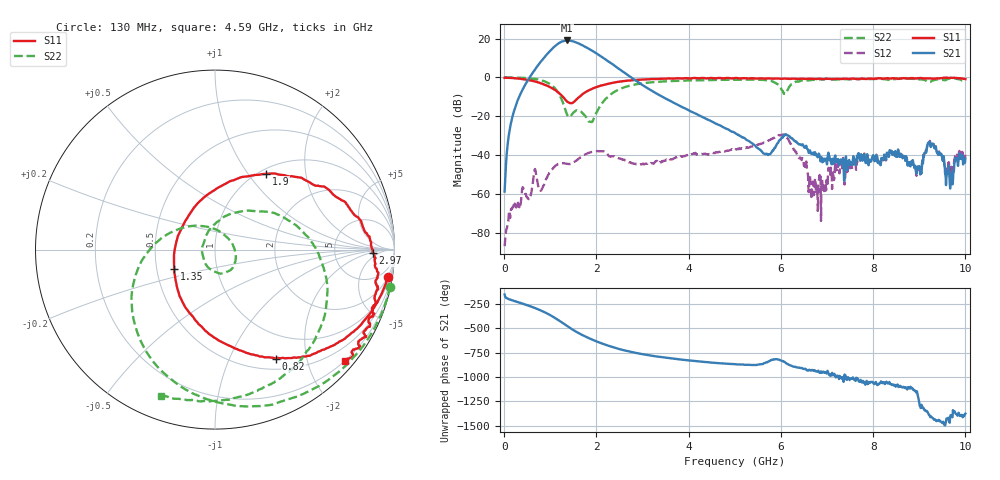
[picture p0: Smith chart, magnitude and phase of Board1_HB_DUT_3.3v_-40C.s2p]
! Created Tue May 27 11:37:13 2025
# hz S ma R 50
! 2 Port Network Data from SP1.SP block
! freq  magS11  angS11  magS21  angS21  magS12  angS12  magS22  angS22
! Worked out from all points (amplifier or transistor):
!   1000 points, 10 MHz to 10 GHz, reference 50 ohm
!   highest |S21| = 19.0 dB at 1.36 GHz (marker M1)
!   |S21| within 3 dB of that: 1.097 GHz to 1.738 GHz (640.7 MHz wide, 45.2 % of centre)
!   unconditionally stable (mu >= 1): 19.38 MHz to 24.58 MHz; 87.49 MHz to 108.8 MHz; 111.2 MHz to end of sweep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
!   at 1.67 GHz: K = 6.85, MAG = 17.5 dB, |S12| = -40.8 dB
!   at 5.01 GHz: K = 11.66, MAG = -9.4 dB, |S12| = -37.1 dB
!   at 10 GHz: K = 402.10, MAG = -30.0 dB, |S12| = -39.7 dB
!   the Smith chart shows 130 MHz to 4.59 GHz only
!   S11 on the Smith chart (normalised r, x): 130 MHz: 2, -12; 820 MHz: 0.64, -1.51; 1.35 GHz: 0.62, -0.14; 1.9 GHz: 1.08, +1.23; 2.97 GHz: 15, -3; 4.59 GHz: 0.20, -2.70
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1e7  0.9781 -1.0  0.001168 -153.1  4.626e-05 65.6  1.005 -0.8
1.3e8  0.9745 -9.2  0.05256 155.9  0.0002452 88.4  0.9983 -12.0
5.6e8  0.8452 -39.4  1.045 88.2  0.0008139 116.0  0.9475 -55.9
8.2e8  0.6952 -60.8  2.755 37.7  0.001361 106.6  0.838 -92.2
9.7e8  0.5825 -75.4  4.47 3.1  0.003342 118.1  0.7077 -119.8
1.12e9  0.4647 -95.0  6.667 -38.3  0.00548 99.2  0.4993 -156.3
1.25e9  0.3432 -121.9  8.355 -79.3  0.006306 81.3  0.2668 159.4
1.35e9  0.2515 -154.5  8.914 -111.9  0.006054 73.1  0.1228 99.0
1.36e9  0.2442 -159.1  8.944 -115.1  0.00606 72.7  0.1143 90.3
1.51e9  0.2334 131.7  8.377 -160.8  0.006617 77.1  0.1276 -25.9
1.68e9  0.3555 84.4  6.875 154.7  0.009294 71.0  0.1272 -85.6
1.9e9  0.5106 55.8  4.924 106.0  0.01218 47.8  0.07153 157.0
2.23e9  0.6764 31.8  2.719 45.8  0.01123 3.9  0.3007 45.8
2.55e9  0.7944 14.9  1.479 0.1  0.007965 -1.1  0.5293 6.3
2.97e9  0.8816 -1.3  0.6721 -42.9  0.005829 10.4  0.7014 -28.3
3.34e9  0.9205 -12.5  0.3655 -71.0  0.006404 13.3  0.7754 -51.2
4.59e9  0.9534 -40.4  0.06455 -134.8  0.012 1.7  0.8659 -110.1
5.01e9  0.972 -48.1  0.03699 -149.5  0.01398 -8.4  0.8754 -126.5
6.07e9  0.9375 -70.0  0.03154 -123.3  0.03293 -98.8  0.3996 -159.0
6.67e9  0.9227 -87.4  0.01079 151.9  0.001225 -149.6  0.8705 -155.8
8.34e9  0.9416 -134.0  0.009171 15.8  0.009149 9.4  0.8664 164.1
1e10  0.9089 -164.1  0.00825 64.5  0.01034 62.2  0.7786 128.4
